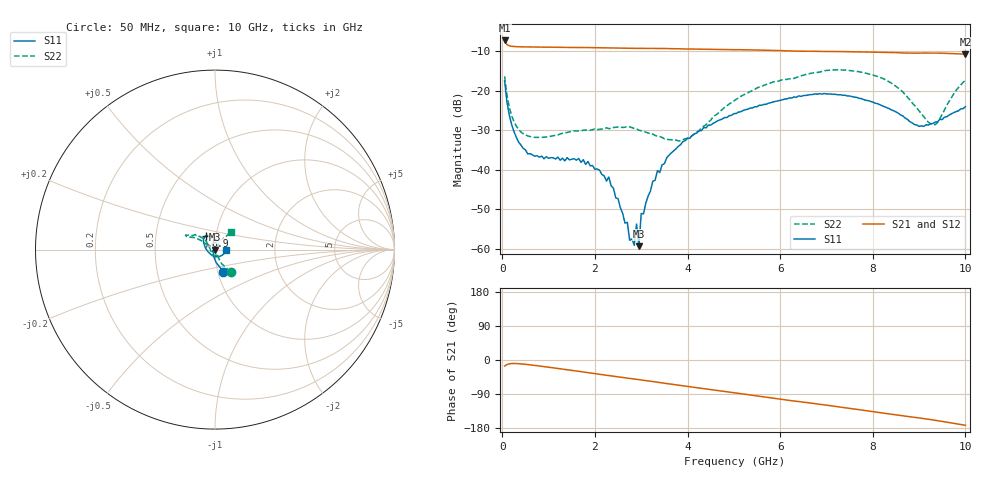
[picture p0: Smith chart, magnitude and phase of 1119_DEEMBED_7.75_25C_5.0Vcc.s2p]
!Hittite Microwave Corp.
!Digital Attenuator/PhaseShifter Rev 1.4.0
!Filename: C:\DATA\DATA\1119_DEEMBED_7.75_25C_5.0Vcc.s2p
!VNA ID: Agilent Technologies,N5224A,MY51441122,A.10.45.03
!Device type:
!2 Port Calibration.
!Temp(C): 25
!Lot Number:
!Serial Number:
!Operator:
!Misc:
!Attenuator:  7.750
# GHZ S DB R 50.0
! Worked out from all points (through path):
!   200 points, 50 MHz to 10 GHz, reference 50 ohm
!   highest |S21| = -7.31 dB at 50 MHz (marker M1); lowest = -10.8 dB at 10 GHz (marker M2)
!   group delay of S21, straight-line fit = 46.3 ps
!   lowest |S11| = -59.3 dB at 2.95 GHz (marker M3), VSWR 1.00, Z = 50.1 - j0.065 ohm
!   |S11| at or under -10 dB: start of sweep to end of sweep
!   |S22| runs from -32.7 to -14.8 dB; largest |S21 - S12| = 0.0015
!   S11 on the Smith chart (normalised r, x): 50 MHz: 1.06, -0.27; 6.9 GHz: 0.89, +0.14; 10 GHz: 1.13, -0.01
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0.05  -17.54 -69.1  -7.31 -16.0  -7.31 -16.0  -16.37 -54.6
0.2  -28.51 -100.2  -8.78 -9.3  -8.78 -9.4  -26.26 -67.0
0.55  -35.96 -130.1  -8.96 -12.0  -8.96 -12.1  -31.43 -61.4
1.75  -37.43 -150.9  -9.10 -31.6  -9.10 -31.6  -29.99 -78.6
2.3  -41.80 -155.4  -9.19 -41.0  -9.20 -41.2  -29.58 -92.3
2.7  -53.25 -98.0  -9.28 -47.6  -9.30 -47.8  -29.10 -102.0
2.75  -57.79 -132.5  -9.29 -48.4  -9.31 -48.6  -29.13 -104.7
2.85  -59.06 -69.8  -9.30 -50.1  -9.32 -50.3  -29.57 -109.2
2.9  -53.68 -6.3  -9.31 -50.9  -9.33 -51.0  -29.65 -113.0
2.95  -59.28 -36.7  -9.30 -51.6  -9.32 -51.8  -29.97 -114.6
3  -51.05 20.8  -9.30 -52.6  -9.32 -52.7  -30.15 -116.5
3.35  -40.19 38.0  -9.34 -58.5  -9.35 -58.6  -31.51 -128.7
3.4  -40.69 45.2  -9.34 -59.4  -9.35 -59.5  -31.59 -131.9
3.55  -36.97 50.2  -9.35 -62.1  -9.36 -62.2  -32.28 -138.6
4.05  -32.01 47.9  -9.47 -70.5  -9.48 -70.6  -31.80 178.7
5.05  -25.76 75.2  -9.65 -87.2  -9.67 -87.2  -22.19 135.7
6.7  -20.97 120.1  -10.04 -114.4  -10.07 -114.5  -15.53 150.9
6.9  -20.85 123.5  -10.08 -117.5  -10.11 -117.6  -15.14 153.1
8.35  -24.52 162.2  -10.34 -142.3  -10.35 -142.4  -17.73 149.4
8.999999  -29.02 -136.6  -10.51 -152.9  -10.53 -152.9  -25.10 147.8
9.35  -27.92 -82.9  -10.50 -159.1  -10.53 -159.2  -28.57 100.8
10  -24.04 -3.5  -10.80 -172.3  -10.82 -172.2  -17.39 47.1
